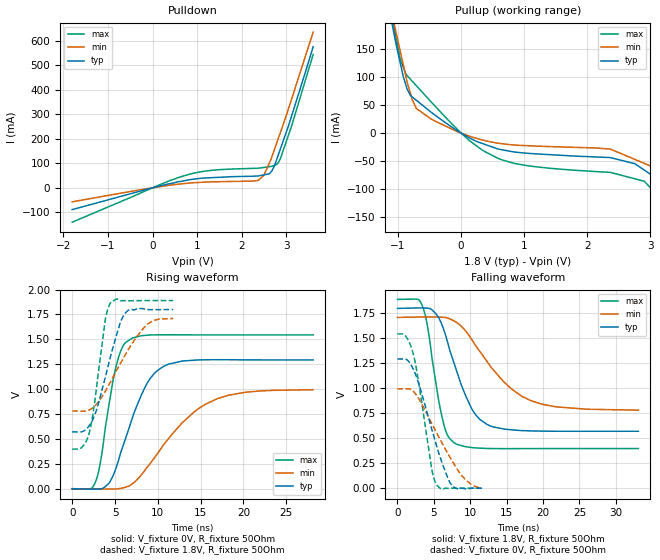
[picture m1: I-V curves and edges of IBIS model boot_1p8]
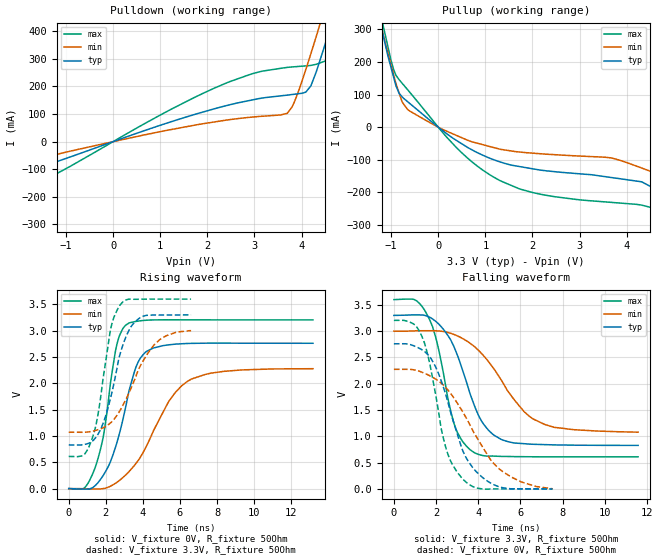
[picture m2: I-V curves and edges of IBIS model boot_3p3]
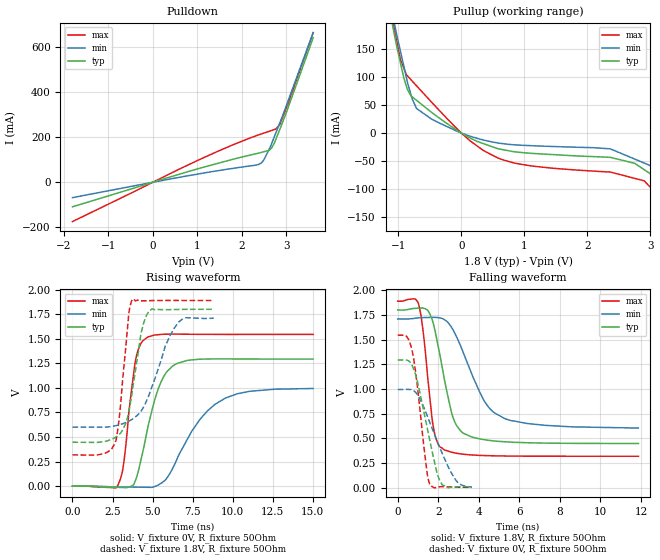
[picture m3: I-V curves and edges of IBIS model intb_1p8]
| Texas Instruments Incorporated
| MCPC Compatible USB Port Multimedia Switch Supports USB, UART, Audio, ID, MIC,
| and Load Switch
| Marketing part#   Digital Voltage Range   Package-type   #pins
| TSU6721YFP   1.65V - 3.6V   WCSP   21
[IBIS Ver]   4.1
[File name]   tsu6721.ibs
[File Rev]   1.0
[Date]   01/10/2013
[Source]
| Texas Instruments Incorporated.
| Analog-eLab Design Center, HPA
| 12500 TI Blvd
| Dallas, TX -75243
| e-mail: elab_scm_ibis@list.ti.com
[Notes]   Revision History:
| Rev 1.0: 01/10/2013
| - Initial version of the model
| - Model generated from simulations in TISPICE
| - Model matched to SPICE simulation
| - C_comp although listed in numerical order of value are
|   obtained from varying PVT conditions. For PVT conditions for
|   each specific value refer the buffer description under
|   respective [Model]. IBIS model user is responsible for using
|   appropriate C_comp to simulate for Signal Integrity.
| - Model names with a trailing _1p8 contains the model for
|   1.8V [1.71V and 1.89V].Model names with a trailing _3p3
|   contains the model for 3.3V [3.0V and 3.6V].
| - Model name jig contains the model for 3.3V [3.0V and 3.6V].
[Disclaimer]
| This model is designed as an aid for customers of Texas Instruments.
| TI and its licensors and suppliers make no warranties, either expressed
| or implied, with respect to this  model, including the warranties of
| merchantability or fitness for a particular purpose. The model is
| provided solely on an "as is" basis. The entire risk as to its quality
| and performance is with the customer.
[Copyright]
(C) Copyright 2013 Texas Instruments Incorporated.All rights reserved.
|   TSU6721
[Component]   TSU6721
[Manufacturer]   TI
[Package]   |21 BGA   -  YSP package
|   typ   min   max
R_pkg   0.005   0.005   0.005
L_pkg   0.2nH   0.2nH   0.2nH
C_pkg   0.6pF   0.6pF   0.6pF
[Pin]  signal_name  model_name   R_pin   L_pin   C_pin
A1   INTB   INTB   0.005   0.2nH   0.6pF
A2   VDDIO   POWER   0.005   0.2nH   0.6pF
A3   ISET   TERM   0.005   0.2nH   0.6pF
A4   OUT   TERM   0.005   0.2nH   0.6pF
A5   VBUS   TERM   0.005   0.2nH   0.6pF
B1   DP_HT   TERM   0.005   0.2nH   0.6pF
B2   SDA   SDA   0.005   0.2nH   0.6pF
B3   S_L   TERM   0.005   0.2nH   0.6pF
B4   MIC   TERM   0.005   0.2nH   0.6pF
B5   DM   TERM   0.005   0.2nH   0.6pF
C1   DM_HT   TERM   0.005   0.2nH   0.6pF
C2   SCL   SCL   0.005   0.2nH   0.6pF
C3   VBUS_CAP   TERM   0.005   0.2nH   0.6pF
C4   S_R   TERM   0.005   0.2nH   0.6pF
C5   DP   TERM   0.005   0.2nH   0.6pF
D1   VBAT   POWER   0.005   0.2nH   0.6pF
D2   IDBP   TERM   0.005   0.2nH   0.6pF
D3   GND   GND   0.005   0.2nH   0.6pF
D4   GND   GND   0.005   0.2nH   0.6pF
D5   ID   TERM   0.005   0.2nH   0.6pF
E1   RxD   TERM   0.005   0.2nH   0.6pF
E2   TxD   TERM   0.005   0.2nH   0.6pF
E3   BOOT   BOOT   0.005   0.2nH   0.6pF
E4   JIG   jig   0.005   0.2nH   0.6pF
E5   GND   GND   0.005   0.2nH   0.6pF
|   Model Selectors
[Model Selector] BOOT
boot_1p8  1.8V digital output
boot_3p3  3.3V digital output
[Model Selector] INTB
intb_1p8  1.8V digital output
intb_3p3  3.3V digital output
[Model Selector] SCL
scl_1p8  1.8V digital input
scl_3p3  3.3V digital input
[Model Selector] SDA
sda_1p8  1.8V digital I/O_open_drain
sda_3p3  3.3V digital I/O_open_drain
[Model Selector] TERM
term_1-8V  1.8V nominal termination
term_3-3V  3.3V nominal termination
[Model] term_1-8V
Model_type Terminator
C_comp   1.0e-20F  1.0e-20F  1.0e-20F
|   typ   min   max
[Voltage Range]   1.8V   1.71V   1.89V
[POWER Clamp Reference]   1.8V   1.71V   1.89V
[GND Clamp Reference]   0V   0V   0V
|Ambient Temperature   25   85   -40
|Junction Temperature
[Temperature Range]   27   125   -40
[Model] term_3-3V
Model_type Terminator
C_comp   1.0e-20F  1.0e-20F  1.0e-20F
|   typ   min   max
[Voltage Range]   3.3V   3.0V   3.6V
[POWER Clamp Reference]   3.3V   3.0V   3.6V
[GND Clamp Reference]   0V   0V   0V
|Ambient Temperature   25   85   -40
|Junction Temperature
[Temperature Range]   27   125   -40
| Models and submodels in the file (11): boot_1p8 (Output), boot_3p3 (Output), intb_1p8 (Output), intb_3p3 (Output), scl_1p8 (Input), scl_3p3 (Input), sda_1p8 (I/O_open_drain), sda_3p3 (I/O_open_drain), jig (Open_drain), term_1-8V (Terminator), term_3-3V (Terminator)
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|   boot_1p8 Model
[Model]   boot_1p8
Model_type   Output
Polarity   Non-Inverting
Vmeas = 0.9
Vref = 0.9
Cref = 2pF
Rref = 50
|   typ   min   max
C_comp   2.622e-12   2.523e-12   2.780e-12
[Voltage Range]   1.8   1.71   1.89
|Ambient Temperature   25   85   -40
|Junction Temperature
[Temperature Range]   27   125   -40
[Pullup Reference]   1.8   1.71   1.89
[Pulldown Reference]   0   0   0
[Power Clamp Reference]   1.8   1.71   1.89
[GND Clamp Reference]   0   0   0
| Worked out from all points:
|   slope of the pulldown table from 0 to 0.27 V, typ, clamps not added: 21.9 ohm
|   slope of the pullup table from 0 to 0.27 V, typ, clamps not added: 17.1 ohm
|   falling waveform, V_fixture 1.8V, R_fixture 50Ohm: 20-80 % time 3.55ns typ, 6.3ns min, 1.99ns max; typ from 1.8 V to 0.571 V
|   rising waveform, V_fixture 0V, R_fixture 50Ohm: 20-80 % time 3.29ns typ, 6.02ns min, 1.76ns max; typ from 0 V to 1.29 V
|   rising waveform, V_fixture 1.8V, R_fixture 50Ohm: 20-80 % time 2.29ns typ, 3.75ns min, 1.39ns max; typ from 0.571 V to 1.8 V
|   falling waveform, V_fixture 0V, R_fixture 50Ohm: 20-80 % time 3.13ns typ, 4.48ns min, 1.97ns max; typ from 1.29 V to 0.001 V
[Pulldown]
|   Voltage   I(typ)   I(min)   I(max)
-1.8V     -89.09mA   -57.32mA   -140.5mA
667.2mV   27.06mA    16.49mA    46.87mA
1.382V    41.83mA    24.37mA    72.36mA
2.367V    48.17mA    30.09mA    79.92mA
2.493V    52.63mA    50.39mA    83.13mA
2.615V    56.94mA    100.4mA    86.22mA
2.673V    68.71mA    125.6mA    88.12mA
2.74V     93.32mA    160.3mA    91.66mA
2.81V     130.1mA    197.1mA    100.4mA
2.865V    158.5mA    225.7mA    118.9mA
3.117V    293.4mA    362.3mA    252.4mA
3.6V      576.3mA    636mA      544.7mA
[Pullup]
|   Voltage   I(typ)   I(min)   I(max)
-1.8V     622.4mA    623.8mA    653.3mA
-1.149V   226.5mA    244.6mA    236mA
-1.026V   156.1mA    176.7mA    166.7mA
-962mV    123.8mA    144.7mA    130.9mA
-856.8mV  78.58mA    92.12mA    102.6mA
-709.7mV  58.52mA    43.88mA    84.53mA
-68.4mV   4.853mA    3.132mA    7.616mA
368.5mV   -19.76mA   -13.06mA   -32.51mA
846.7mV   -33.66mA   -21.18mA   -54.05mA
2.362V    -43.62mA   -28.38mA   -69.99mA
2.901V    -65.74mA   -53.84mA   -85.74mA
3.6V      -119.6mA   -86.88mA   -168.1mA
[Ramp]
R_load = 50
|   typ   min   max
dV/dt_r   0.775996/3.28238e-09   0.597035/6.02547e-09   0.926799/1.76372e-09
dV/dt_f   0.737495/3.54751e-09   0.557745/6.26787e-09   0.895355/1.9821e-09
[Falling Waveform]
V_fixture = 1.8V
V_fixture_min = 1.71V
V_fixture_max = 1.89V
R_fixture = 50Ohm
|   Time   V(typ)   V(min)   V(max)
0s        1.8V       1.71V      1.89V
3.375ns   1.805V     1.714V     1.834V
4.1ns     1.803V     1.714V     1.635V
6.175ns   1.625V     1.711V     699.2mV
7.825ns   1.242V     1.673V     453.3mV
10.3ns    784.4mV    1.479V     406.8mV
13.05ns   615.6mV    1.197V     397.8mV
16.98ns   577.7mV    926mV      397.1mV
19.88ns   572mV      841.1mV    397.5mV
33.1ns    570.8mV    781.8mV    397.7mV
[Rising Waveform]
V_fixture = 0V
V_fixture_min = 0V
V_fixture_max = 0V
R_fixture = 50Ohm
|   Time   V(typ)   V(min)   V(max)
0s        2.608nV    187nV      110.6pV
2.725ns   -4.619mV   -3.218mV   69.05mV
3.35ns    -2.727mV   -3.453mV   290.9mV
5.1ns     202mV      -2.356mV   1.219V
5.875ns   414.3mV    7.436mV    1.423V
6.75ns    637.6mV    32.71mV    1.499V
8.825ns   1.07V      223mV      1.543V
11.3ns    1.253V     508.8mV    1.546V
16.95ns   1.296V     904.2mV    1.545V
28.15ns   1.293V     994.5mV    1.545V
[Rising Waveform]
V_fixture = 1.8V
V_fixture_min = 1.71V
V_fixture_max = 1.89V
R_fixture = 50Ohm
|   Time   V(typ)   V(min)   V(max)
0s        570.8mV    780.4mV    397.7mV
1.125ns   571.7mV    779mV      416.1mV
1.975ns   630.7mV    790.1mV    556.4mV
2.575ns   728.7mV    825.6mV    839mV
3.85ns    1.114V     976.3mV    1.689V
4.45ns    1.32V      1.07V      1.864V
5.65ns    1.678V     1.261V     1.888V
6.5ns     1.789V     1.39V      1.888V
8.8ns     1.798V     1.654V     1.89V
11.8ns    1.8V       1.71V      1.89V
[Falling Waveform]
V_fixture = 0V
V_fixture_min = 0V
V_fixture_max = 0V
R_fixture = 50Ohm
|   Time   V(typ)   V(min)   V(max)
0s        1.293V     995.1mV    1.545V
1.1ns     1.293V     996.1mV    1.525V
2.175ns   1.193V     971.1mV    1.343V
2.8ns     1.075V     912.3mV    1.113V
4.75ns    582.7mV    643.7mV    175.5mV
5.325ns   439.2mV    562.6mV    42.56mV
6.8ns     126.1mV    363.7mV    -403.5uV
7.675ns   15.5mV     255.2mV    1.481mV
9.5ns     -5.302mV   75.91mV    435.5uV
11.6ns    998uV      -1.689mV   40.39uV
|   boot_3p3 Model
[Model]   boot_3p3
Model_type   Output
Polarity   Non-Inverting
Vmeas = 1.65
Vref = 1.65
Cref = 2pF
Rref = 50
|   typ   min   max
C_comp   2.588e-12   2.461e-12   2.799e-12
[Voltage Range]   3.3   3   3.6
|Ambient Temperature   25   85   -40
|Junction Temperature
[Temperature Range]   27   125   -40
[Pullup Reference]   3.3   3   3.6
[Pulldown Reference]   0   0   0
[Power Clamp Reference]   3.3   3   3.6
[GND Clamp Reference]   0   0   0
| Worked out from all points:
|   slope of the pulldown table from 0 to 0.495 V, typ, clamps not added: 16.6 ohm
|   slope of the pullup table from 0 to 0.495 V, typ, clamps not added: 9.78 ohm
|   falling waveform, V_fixture 3.3V, R_fixture 50Ohm: 20-80 % time 1.38ns typ, 2.13ns min, 986ps max; typ from 3.3 V to 0.828 V
|   rising waveform, V_fixture 0V, R_fixture 50Ohm: 20-80 % time 1.24ns typ, 2.16ns min, 866ps max; typ from 0 V to 2.76 V
|   rising waveform, V_fixture 3.3V, R_fixture 50Ohm: 20-80 % time 1.06ns typ, 1.63ns min, 774ps max; typ from 0.829 V to 3.3 V
|   falling waveform, V_fixture 0V, R_fixture 50Ohm: 20-80 % time 1.38ns typ, 2.11ns min, 986ps max; typ from 2.76 V to 0.001 V
[Pulldown]
|   Voltage   I(typ)   I(min)   I(max)
-3.3V     -197.4mA   -130mA     -309.5mA
1.782V    101.2mA    61.31mA    164.7mA
2.934V    150.4mA    88.7mA     245mA
3.69V     168.4mA    102.3mA    268.9mA
3.855V    171.9mA    147mA      271.3mA
4.089V    179.2mA    261mA      274.3mA
4.198V    202.1mA    318.9mA    276.2mA
4.316V    255.2mA    384.1mA    280.4mA
4.468V    336mA      469.4mA    289.9mA
4.572V    395.1mA    528.4mA    313.6mA
4.824V    540.8mA    673.9mA    447.6mA
6.6V      1.633A     1.734A     1.567A
[Pullup]
|   Voltage   I(typ)   I(min)   I(max)
-3.3V     1.653A     1.594A     1.765A
-1.217V   311mA      313.2mA    342.1mA
-1.125V   254.1mA    258.9mA    283.6mA
-894.3mV  125.5mA    132.3mA    158.4mA
-648mV    77.92mA    53.78mA    114.6mA
478.8mV   -49.17mA   -31.17mA   -75.98mA
1.318V    -106.9mA   -68mA      -164.6mA
3.702V    -155.2mA   -95.49mA   -231.2mA
4.316V    -167.7mA   -125.4mA   -239.2mA
4.892V    -214.4mA   -156.9mA   -284.1mA
6V        -306.6mA   -217.8mA   -427.4mA
6.6V      -356.6mA   -250.8mA   -505mA
[Ramp]
R_load = 50
|   typ   min   max
dV/dt_r   1.65636/1.24105e-09   1.36482/2.15966e-09   1.92298/8.64266e-10
dV/dt_f   1.48248/1.37998e-09   1.15775/2.13974e-09   1.79319/9.80518e-10
[Falling Waveform]
V_fixture = 3.3V
V_fixture_min = 3V
V_fixture_max = 3.6V
R_fixture = 50Ohm
|   Time   V(typ)   V(min)   V(max)
0s        3.3V       3V         3.6V
950ps     3.31V      3.005V     3.604V
1.575ns   3.286V     3.009V     3.314V
2.025ns   3.173V     3.006V     2.816V
2.875ns   2.678V     2.934V     1.215V
3.775ns   1.629V     2.722V     699.7mV
4.775ns   1.015V     2.264V     623.8mV
6.6ns     849.5mV    1.331V     611.8mV
7.625ns   837.7mV    1.17V      610.8mV
11.57ns   828.3mV    1.08V      611.2mV
[Rising Waveform]
V_fixture = 0V
V_fixture_min = 0V
V_fixture_max = 0V
R_fixture = 50Ohm
|   Time   V(typ)   V(min)   V(max)
0s        5.863nV    303.6nV    247pV
875ps     -10.48mV   -4.738mV   22.96mV
1.45ns    64.61mV    -8.639mV   424.5mV
1.875ns   259.2mV    978.2uV    1.011V
2.55ns    816.9mV    107.3mV    2.664V
3.075ns   1.556V     260.5mV    3.104V
4.15ns    2.593V     777.6mV    3.197V
5.4ns     2.731V     1.658V     3.207V
6.625ns   2.759V     2.082V     3.206V
13.18ns   2.761V     2.277V     3.205V
[Rising Waveform]
V_fixture = 3.3V
V_fixture_min = 3V
V_fixture_max = 3.6V
R_fixture = 50Ohm
|   Time   V(typ)   V(min)   V(max)
0s        829.2mV    1.07V      611.4mV
800ps     835.1mV    1.07V      637.9mV
1.25ns    893.6mV    1.089V     937.9mV
1.6ns     1.047V     1.121V     1.455V
2.25ns    1.71V      1.247V     3.014V
2.775ns   2.561V     1.489V     3.489V
3.45ns    3.119V     1.979V     3.595V
4.6ns     3.299V     2.726V     3.6V
5.275ns   3.297V     2.905V     3.6V
6.6ns     3.3V       3V         3.6V
[Falling Waveform]
V_fixture = 0V
V_fixture_min = 0V
V_fixture_max = 0V
R_fixture = 50Ohm
|   Time   V(typ)   V(min)   V(max)
0s        2.761V     2.275V     3.205V
900ps     2.728V     2.268V     3.145V
1.3ns     2.654V     2.224V     2.927V
1.675ns   2.524V     2.158V     2.427V
2.25ns    2.05V      2.008V     1.133V
2.475ns   1.769V     1.922V     768.3mV
3.275ns   717.3mV    1.457V     185.1mV
3.925ns   320.1mV    982.5mV    17.74mV
5ns       39.81mV    378.8mV    343.7uV
7.525ns   891.7uV    3.317mV    -88.96uV
|   intb_1p8 Model
[Model]   intb_1p8
Model_type   Output
Polarity   Non-Inverting
Vmeas = 0.9
Vref = 0.9
Cref = 2pF
Rref = 50
|   typ   min   max
C_comp   2.656e-12   2.539e-12   2.894e-12
[Voltage Range]   1.8   1.71   1.89
|Ambient Temperature   25   85   -40
|Junction Temperature
[Temperature Range]   27   125   -40
[Pullup Reference]   1.8   1.71   1.89
[Pulldown Reference]   0   0   0
[Power Clamp Reference]   1.8   1.71   1.89
[GND Clamp Reference]   0   0   0
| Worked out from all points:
|   slope of the pulldown table from 0 to 0.27 V, typ, clamps not added: 16.4 ohm
|   slope of the pullup table from 0 to 0.27 V, typ, clamps not added: 17.1 ohm
|   falling waveform, V_fixture 1.8V, R_fixture 50Ohm: 20-80 % time 818ps typ, 1.46ns min, 485ps max; typ from 1.8 V to 0.447 V
|   rising waveform, V_fixture 0V, R_fixture 50Ohm: 20-80 % time 1.2ns typ, 2.32ns min, 635ps max; typ from 0 V to 1.29 V
|   rising waveform, V_fixture 1.8V, R_fixture 50Ohm: 20-80 % time 792ps typ, 1.47ns min, 541ps max; typ from 0.447 V to 1.8 V
|   falling waveform, V_fixture 0V, R_fixture 50Ohm: 20-80 % time 795ps typ, 1.19ns min, 515ps max; typ from 1.29 V to 0.007 V
[Pulldown]
|   Voltage   I(typ)   I(min)   I(max)
-1.8V     -108.7mA   -68.08mA   -174.3mA
1.058V    62.45mA    38.17mA    101.6mA
2.291V    125.6mA    75.46mA    204.4mA
2.432V    132.3mA    84.96mA    214.2mA
2.488V    135.3mA    97.67mA    218mA
2.615V    142mA      148.1mA    226.5mA
2.669V    153mA      172.4mA    230.1mA
2.729V    174.2mA    202.3mA    234.1mA
2.761V    190.3mA    218.7mA    236.3mA
2.846V    232.8mA    261.5mA    255.1mA
3.026V    325.1mA    355.5mA    343.1mA
3.6V      641.9mA    664.4mA    663.7mA
[Pullup]
|   Voltage   I(typ)   I(min)   I(max)
-1.8V     622.4mA    623.8mA    653.3mA
-1.149V   226.5mA    244.6mA    236mA
-1.026V   156.1mA    176.7mA    166.7mA
-962mV    123.8mA    144.7mA    130.9mA
-856.8mV  78.58mA    92.12mA    102.6mA
-709.7mV  58.52mA    43.88mA    84.53mA
-68.4mV   4.853mA    3.132mA    7.616mA
368.5mV   -19.76mA   -13.06mA   -32.51mA
846.7mV   -33.66mA   -21.18mA   -54.05mA
2.362V    -43.62mA   -28.38mA   -69.99mA
2.901V    -65.74mA   -53.84mA   -85.74mA
3.6V      -119.6mA   -86.88mA   -168.1mA
[Ramp]
R_load = 50
|   typ   min   max
dV/dt_r   0.775996/1.20048e-09   0.597034/2.30975e-09   0.926799/6.34557e-10
dV/dt_f   0.811663/8.17786e-10   0.665519/1.46261e-09   0.943136/4.84351e-10
[Falling Waveform]
V_fixture = 1.8V
V_fixture_min = 1.71V
V_fixture_max = 1.89V
R_fixture = 50Ohm
|   Time   V(typ)   V(min)   V(max)
0s        1.8V       1.71V      1.89V
1.025ns   1.819V     1.721V     1.864V
1.275ns   1.819V     1.724V     1.549V
1.775ns   1.649V     1.726V     594.8mV
2.275ns   1.129V     1.706V     386.4mV
2.675ns   746.8mV    1.619V     358.5mV
3.05ns    590.3mV    1.462V     343.5mV
4.25ns    486.9mV    884.5mV    325.4mV
4.9ns     470.5mV    742.9mV    321.9mV
11.88ns   447.3mV    603.8mV    318.1mV
[Rising Waveform]
V_fixture = 0V
V_fixture_min = 0V
V_fixture_max = 0V
R_fixture = 50Ohm
|   Time   V(typ)   V(min)   V(max)
0s        88.42pV    245.9pV    63.06pV
2.85ns    -12.38mV   -8.316mV   14.01mV
3.2ns     -14.32mV   -8.905mV   236.5mV
3.925ns   54.36mV    -10.03mV   1.271V
4.675ns   574mV      -11.7mV    1.515V
5.525ns   1.06V      28.49mV    1.544V
6.525ns   1.248V     275.8mV    1.548V
7.975ns   1.292V     682.2mV    1.545V
9.55ns    1.295V     896.9mV    1.545V
15.03ns   1.293V     994mV      1.545V
[Rising Waveform]
V_fixture = 1.8V
V_fixture_min = 1.71V
V_fixture_max = 1.89V
R_fixture = 50Ohm
|   Time   V(typ)   V(min)   V(max)
0s        447.2mV    600.8mV    318.1mV
1.95ns    452.8mV    600mV      331.3mV
2.7ns     498.3mV    615.5mV    459.5mV
2.95ns    531.9mV    626mV      742.9mV
3.525ns   765.6mV    662.3mV    1.77V
3.75ns    984.1mV    683mV      1.902V
4.3ns     1.568V     767.1mV    1.886V
4.825ns   1.789V     949.4mV    1.888V
6.6ns     1.799V     1.665V     1.89V
8.817ns   1.8V       1.71V      1.89V
[Falling Waveform]
V_fixture = 0V
V_fixture_min = 0V
V_fixture_max = 0V
R_fixture = 50Ohm
|   Time   V(typ)   V(min)   V(max)
0s        1.293V     995.1mV    1.545V
450ps     1.292V     996mV      1.53V
725ps     1.232V     988.2mV    1.375V
925ps     1.111V     955.8mV    1.104V
1.45ns    610.4mV    731.9mV    151.6mV
1.6ns     462.8mV    651.8mV    26.86mV
1.95ns    140.6mV    469.3mV    8.662mV
2.2ns     30.92mV    345.4mV    9.848mV
2.9ns     7.615mV    67.2mV     5.528mV
3.65ns    6.754mV    8.352mV    2.879mV
